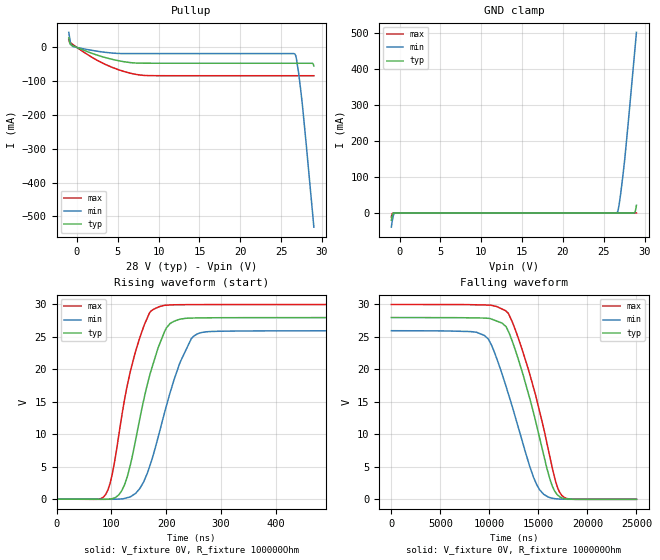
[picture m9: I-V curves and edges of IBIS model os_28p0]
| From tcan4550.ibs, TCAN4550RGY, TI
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|   os_28p0 Model
[Model]   os_28p0
Model_type   Open_source
Polarity   Non-Inverting
Vmeas = 14
Vref = 0
Cref = 2pF
Rref = 100000
|   typ   min   max
C_comp   1.264pF   1.235pF   1.281pF
|  Where Nom  PVT is Nominal Process, 28V,   27C
|   Fast PVT is Strong Process,  30V, -40C
|   Slow PVT is Weak Process,   26V, 150C
[Voltage Range]   28   26   30
|Junction Temperature
[Temperature Range]   27   150   -40
[Pullup Reference]   28   26   30
[Pulldown Reference]   0   0   0
[Power Clamp Reference]   28   26   30
[GND Clamp Reference]   0   0   0
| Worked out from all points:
|   slope of the pullup table from 0 to 4.2 V, typ, clamps not added: 122 ohm
|   GND clamp passes 1 mA (typ) near -0.80 V on its own axis
|   falling waveform, V_fixture 0V, R_fixture 100000Ohm: 20-80 % time 2.96us typ, 3.13us min, 3.12us max; typ from 28 V to 0 V
|   rising waveform, V_fixture 0V, R_fixture 100000Ohm: 20-80 % time 46.2ns typ, 53.6ns min, 42.2ns max; typ from 0 V to 28 V
[GND Clamp]
|   Voltage   I(typ)   I(min)   I(max)
-1V       -20.26mA   -39.39mA   -11.19mA
-880mV    -5.343mA   -20.85mA   -1.172mA
-760mV    -316.1uA   -7.462mA   -180.2uA
-580mV    -1.77uA    -285.6uA   -2.131uA
26.63V    42.68nA    1.102mA    38.94nA
26.75V    43.05nA    7.63mA     39.05nA
26.9V     43.57nA    25.98mA    39.19nA
27.35V    45.77nA    104.7mA    39.69nA
27.56V    47.38nA    147.4mA    39.97nA
28.76V    294uA      441.1mA    42.43nA
28.85V    3.455mA    463.8mA    42.72nA
29V       21.43mA    501.7mA    43.26nA
[Pullup]
|   Voltage   I(typ)   I(min)   I(max)
-1V       28.24mA    44.83mA    23.98mA
-880mV    13.34mA    26.12mA    15.52mA
-760mV    8.1mA      11.67mA    13.24mA
-520mV    5.401mA    2.745mA    9mA
3.47V     -29.85mA   -14.36mA   -50.09mA
7.4V      -46.25mA   -18.11mA   -80.44mA
26.69V    -46.68mA   -19.61mA   -83.67mA
26.84V    -46.68mA   -29.96mA   -83.67mA
27.11V    -46.69mA   -71.06mA   -83.67mA
27.59V    -46.69mA   -168.4mA   -83.67mA
28.82V    -46.81mA   -484.1mA   -83.67mA
29V       -54.67mA   -531.8mA   -83.67mA
[Ramp]
R_load = 100000
|   typ   min   max
dV/dt_r   16.7834/4.62461e-08   15.5691/5.36021e-08   17.9894/4.21937e-08
dV/dt_f   16.7834/2.96212e-06   15.5691/3.12852e-06   17.9894/3.11608e-06
[Falling Waveform]
V_fixture = 0V
V_fixture_min = 0V
V_fixture_max = 0V
R_fixture = 100000Ohm
C_fixture = 0F
|   Time   V(typ)   V(min)   V(max)
0s        27.97V     25.95V     29.98V
9.476us   27.89V     25.23V     29.91V
10.23us   27.73V     23.69V     29.85V
11.67us   26.63V     17.54V     29.02V
12.91us   21.76V     11.29V     24.99V
14.83us   11.31V     2.253V     15.34V
16.41us   2.055V     167.8mV    4.862V
16.96us   656.5mV    62.94mV    1.78V
17.39us   232.3mV    27.97mV    595.2mV
25us      447.4uV    348.6uV    404.7uV
[Rising Waveform]
V_fixture = 0V
V_fixture_min = 0V
V_fixture_max = 0V
R_fixture = 100000Ohm
C_fixture = 0F
|   Time   V(typ)   V(min)   V(max)
0s        461.3uV    351.4uV    404.7uV
89.67ns   -15.63mV   -11.41mV   741.6mV
101.4ns   77.71mV    -11.8mV    3.768V
119ns     1.328V     45.3mV     12.89V
143.9ns   9.025V     880.9mV    22.73V
169.8ns   19.08V     5.075V     28.76V
214.3ns   27.4V      18.44V     29.94V
256.1ns   27.91V     25.43V     29.96V
392.7ns   27.96V     25.92V     29.98V
25us      27.97V     25.95V     29.98V
